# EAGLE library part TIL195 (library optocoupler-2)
TEXAS INSTRUMENTS OPTO COUPLER
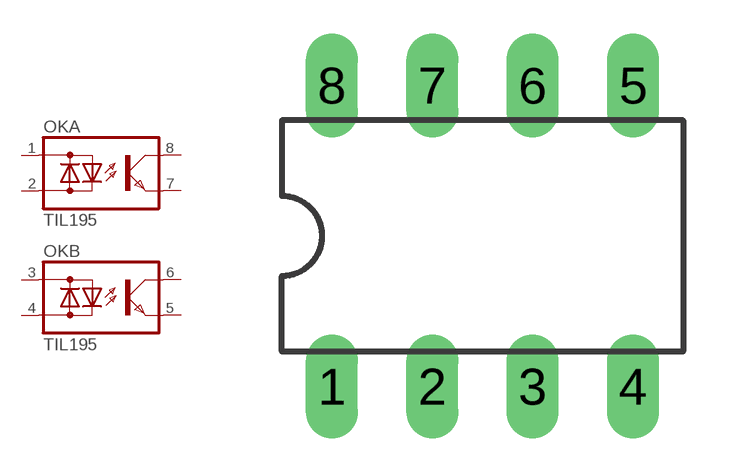
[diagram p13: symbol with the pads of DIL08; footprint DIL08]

Designator prefix OK; gates A=OK-LD B=OK-LD

## TIL195  [DIL08]
1  A:AC1  pas
2  A:AC2  pas
3  B:AC1  pas
4  B:AC2  pas
5  B:E  pas
6  B:C  pas
7  A:E  pas
8  A:C  pas

## Footprint DIL08 (pad centres in mm)
Dual In Line Package
drill 0.813 long: 1 -3.81,-3.81; 2 -1.27,-3.81; 3 1.27,-3.81; 4 3.81,-3.81; 5 3.81,3.81; 6 1.27,3.81; 7 -1.27,3.81; 8 -3.81,3.81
